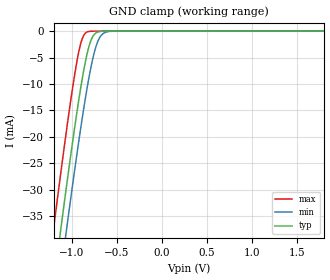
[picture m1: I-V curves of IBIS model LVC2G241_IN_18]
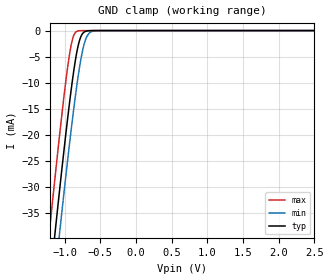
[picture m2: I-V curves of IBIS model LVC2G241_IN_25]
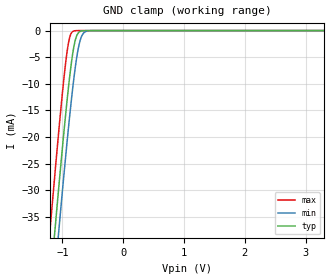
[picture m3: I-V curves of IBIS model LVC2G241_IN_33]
| TEXAS INSTRUMENTS INCORPORATED
| Standard Linear and Logic Group
| IBIS Model of SN74LVC2G241
| Dual Buffer/Driver with 3-State Outputs
| This file contains package information for the following:
|  TSSOP 8-pin (DCT) package as [Component] LVC2G241_DCT
|  VSSOP 8-pin (DCU) package as [Component] LVC2G241_DCU
|  NanoStar WCSP 8-pin (YEA) package as [Component] LVC2G241_YEA
|  NanoFree WCSP 8-pin (YZA) package as [Component] LVC2G241_YZA
|  NanoStar WCSP 8-pin (YEP) package as [Component] LVC2G241_YEP
|  NanoFree WCSP 8-pin (YZP) package as [Component] LVC2G241_YZP
| This device can be powered at the following Vccs:
| This device can be powered at the following Vccs:
|  1.8 volt Vcc
|  2.5 volt Vcc
|  3.3 volt Vcc
|  5 volt Vcc
| This file provides unique models under the [Model Selector] for each Vcc.
| For operation at a specific Vcc, select the appropriate model after each
| [Model Selector] keyword.
[IBIS Ver]   3.2
[Comment char]  |_char
[File Name]   sn74lvc2g241.ibs
[File Rev]   1.2 | d_die
[Date]   October 23, 2003
[Source]   Data created from TI-SPICE simulations at TI-SLL.
[Notes]   The following is an IBIS list for the LVC2G241.
   Please contact sllibis@ti.com with questions and
   comments concerning SLL IBIS models.
   -Power clamp data deleted as there is no power-clamp diode.
[Disclaimer] Property of Texas Instruments Incorporated.  Unauthorized
   reproduction and/or distribution is strictly prohibited.
   This product is protected under copyright law.
   Created  2002, (C) Copyright  2002, Texas Instruments
   Incorporated, All Rights Reserved
   UNLESS THERE IS A SIGNED, WRITTEN AGREEMENT TO THE
   CONTRARY, TEXAS INSTRUMENTS (TI) IS PROVIDING THE IBIS
   MODELS  AND WITHOUT ANY WARRANTY, EXPRESSED OR
   IMPLIED.  TI assumes no liability for:
   1) the accuracy of the IBIS models provided to your
   company;
   2) the proper functioning of these IBIS Models in your
   design or for any resulting applications; or
   3) infringement of patents, copyrights or intellectual
   property rights resulting from your use of these IBIS
   models.
   TI provides IBIS Models as a service to our customers.
   You and your company shall not distribute, sell or give
   these models to anyone else without prior written
   permission from TI.
   TI reserves the right to make changes to our products or
   to discontinue any semiconductor product or service
   without notice, and advises our customers to obtain the
   latest version of relevant information to verify, before
   placing orders, that the information being relied on is
   current.
   Please be aware that your receipt and use of the IBIS
   information provided shall serve as acceptance of these
   terms and conditions.  If you do not accept these terms,
   you should return or destroy the IBIS models and any
   other accompanying information immediately.
| Component LVC2G241_DCT 8-pin TSSOP
[Component]   LVC2G241_DCT
[Manufacturer]   Texas Instruments, Inc.
[Package]
|   typ   min   max
R_pkg   2.900e-02   2.800e-02   3.100e-02
L_pkg   1.796e-09   1.666e-09   1.924e-09
C_pkg   1.090e-13   8.300e-14   1.360e-13
[Pin]   signal_name   model_name   R_pin   L_pin   C_pin
1   1NOE   LVC2G241_IN   3.100e-02   1.894e-09   1.340e-13
2   1A   LVC2G241_IN   2.800e-02   1.697e-09   8.600e-14
3   2Y   LVC2G241_OUT   3.000e-02   1.722e-09   8.600e-14
4   GND   GND   3.000e-02   1.861e-09   1.300e-13
5   2A   LVC2G241_IN   2.800e-02   1.924e-09   1.360e-13
6   1Y   LVC2G241_OUT   2.900e-02   1.736e-09   8.600e-14
7   2OE   LVC2G241_IN   2.800e-02   1.666e-09   8.300e-14
8   VCC   POWER   3.000e-02   1.871e-09   1.320e-13
| Component LVC2G241_DCU 8-pin SOT
[Component]   LVC2G241_DCU
[Manufacturer]   Texas Instruments, Inc.
[Package]
|   typ   min   max
R_pkg   2.600e-02   2.300e-02   3.800e-02
L_pkg   1.394e-09   1.066e-09   2.046e-09
C_pkg   2.590e-13   2.150e-13   3.720e-13
[Pin]   signal_name   model_name   R_pin   L_pin   C_pin
1   1NOE   LVC2G241_IN   2.400e-02   1.520e-09   2.710e-13
2   1A   LVC2G241_IN   2.300e-02   1.112e-09   2.180e-13
3   2Y   LVC2G241_OUT   2.300e-02   1.070e-09   2.170e-13
4   GND   GND   2.700e-02   2.046e-09   3.720e-13
5   2A   LVC2G241_IN   2.700e-02   1.542e-09   2.730e-13
6   1Y   LVC2G241_IN   2.300e-02   1.100e-09   2.240e-13
7   2NOE   LVC2G241_OUT   2.300e-02   1.066e-09   2.150e-13
8   VCC   POWER   3.800e-02   1.696e-09   2.800e-13
| Component LVC2G241_YEA 8-pin NanoStar WCSP
[Component]   LVC2G241_YEA
[Manufacturer]   Texas Instruments, Inc.
[Package]
|   typ   min   max
R_pkg   0.001   0.001   0.001
L_pkg   0.021nH   0.021nH   0.021nH
C_pkg   0.043pF   0.042pF   0.044pF
[Pin]   signal_name   model_name   R_pin   L_pin   C_pin
1   1NOE   LVC2G241_IN   0.046   2.861nH   0.321pF
2   1A   LVC2G241_IN   0.037   2.437nH   0.286pF
3   2Y   LVC2G241_OUT   0.034   2.419nH   0.286pF
4   GND   GND   0.043   2.784nH   0.321pF
5   2A   LVC2G241_IN   0.043   2.784nH   0.321pF
6   1Y   LVC2G241_IN   0.035   2.420nH   0.286pF
7   2NOE   LVC2G241_OUT   0.037   2.437nH   0.286pF
8   VCC   POWER   0.046   2.860nH   0.321pF
| Component LVC2G241_YZA 8-pin NanoFree WCSP
[Component]   LVC2G241_YZA
[Manufacturer]   Texas Instruments, Inc.
[Package]
|   typ   min   max
R_pkg   0.001   0.001   0.001
L_pkg   0.021nH   0.021nH   0.021nH
C_pkg   0.043pF   0.042pF   0.044pF
[Pin]   signal_name   model_name   R_pin   L_pin   C_pin
1   1NOE   LVC2G241_IN   0.046   2.861nH   0.321pF
2   1A   LVC2G241_IN   0.037   2.437nH   0.286pF
3   2Y   LVC2G241_OUT   0.034   2.419nH   0.286pF
4   GND   GND   0.043   2.784nH   0.321pF
5   2A   LVC2G241_IN   0.043   2.784nH   0.321pF
6   1Y   LVC2G241_IN   0.035   2.420nH   0.286pF
7   2NOE   LVC2G241_OUT   0.037   2.437nH   0.286pF
8   VCC   POWER   0.046   2.860nH   0.321pF
| Component LVC2G241_YEP 8-pin NanoStar WCSP
[Component]   LVC2G241_YEP
[Manufacturer]   Texas Instruments, Inc.
[Package]
|   typ   min   max
R_pkg   0.001   0.001   0.001
L_pkg   0.021nH   0.021nH   0.021nH
C_pkg   0.043pF   0.042pF   0.044pF
[Pin]   signal_name   model_name   R_pin   L_pin   C_pin
1   1NOE   LVC2G241_IN   0.046   2.861nH   0.321pF
2   1A   LVC2G241_IN   0.037   2.437nH   0.286pF
3   2Y   LVC2G241_OUT   0.034   2.419nH   0.286pF
4   GND   GND   0.043   2.784nH   0.321pF
5   2A   LVC2G241_IN   0.043   2.784nH   0.321pF
6   1Y   LVC2G241_IN   0.035   2.420nH   0.286pF
7   2NOE   LVC2G241_OUT   0.037   2.437nH   0.286pF
8   VCC   POWER   0.046   2.860nH   0.321pF
| Component LVC2G241_YZP 8-pin NanoFree WCSP
[Component]   LVC2G241_YZP
[Manufacturer]   Texas Instruments, Inc.
[Package]
|   typ   min   max
R_pkg   0.001   0.001   0.001
L_pkg   0.021nH   0.021nH   0.021nH
C_pkg   0.043pF   0.042pF   0.044pF
[Pin]   signal_name   model_name   R_pin   L_pin   C_pin
1   1NOE   LVC2G241_IN   0.046   2.861nH   0.321pF
2   1A   LVC2G241_IN   0.037   2.437nH   0.286pF
3   2Y   LVC2G241_OUT   0.034   2.419nH   0.286pF
4   GND   GND   0.043   2.784nH   0.321pF
5   2A   LVC2G241_IN   0.043   2.784nH   0.321pF
6   1Y   LVC2G241_IN   0.035   2.420nH   0.286pF
7   2NOE   LVC2G241_OUT   0.037   2.437nH   0.286pF
8   VCC   POWER   0.046   2.860nH   0.321pF
| Model LVC2G241_IN
[Model Selector]   LVC2G241_IN
LVC2G241_IN_18   1.8 volt Vcc
LVC2G241_IN_25   2.5 volt Vcc
LVC2G241_IN_33   3.3 volt Vcc
LVC2G241_IN_50   5 volt Vcc
| Model LVC2G241_OUT
[Model Selector]   LVC2G241_OUT
LVC2G241_OUT_18   1.8 volt Vcc
LVC2G241_OUT_25   2.5 volt Vcc
LVC2G241_OUT_33   3.3 volt Vcc
LVC2G241_OUT_50   5 volt Vcc
| Models and submodels in the file (8): LVC2G241_IN_18 (Input), LVC2G241_IN_25 (Input), LVC2G241_IN_33 (Input), LVC2G241_IN_50 (Input), LVC2G241_OUT_18 (3-state), LVC2G241_OUT_25 (3-state), LVC2G241_OUT_33 (3-state), LVC2G241_OUT_50 (3-state)
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[Model]   LVC2G241_IN_18
Model_type  Input
Vinl=0.5775
Vinh=1.2675
| variable   typ   min   max
C_comp   3.50pF   2.99pF   4.32pF
[Temperature Range]   40   100   -40
| Ambient temperature   25   85   -40
[Voltage range]   1.8   1.65   1.95
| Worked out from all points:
|   GND clamp passes 1 mA (typ) near -0.77 V on its own axis
[GND Clamp]
| LVC2G241D_IN_18
|   Voltage   I(typ)   I(min)   I(max)
-1.8V     -129.8mA   -137.8mA   -119.7mA
-1.205V   -48.27mA   -56.56mA   -37.63mA
-1.125V   -37.77mA   -46.06mA   -27.13mA
-1.06V    -29.44mA   -37.69mA   -18.89mA
-980mV    -19.61mA   -27.69mA   -9.485mA
-925mV    -13.29mA   -21.11mA   -4.122mA
-880mV    -8.606mA   -15.99mA   -1.263mA
-835mV    -4.656mA   -11.25mA   -214.1uA
-780mV    -1.472mA   -6.227mA   -17.15uA
-725mV    -285.9uA   -2.596mA   -1.294uA
-615mV    -6.479uA   -167.8uA   -7.305nA
1.8V      3.326pA    6.142pA    3.026pA
[Model]   LVC2G241_IN_25
Model_type  Input
Vinl=0.7
Vinh=1.7
| variable   typ   min   max
C_comp   3.42pF   2.80pF   4.39pF
[Temperature Range]   40   100   -40
| Ambient temperature   25   85   -40
[Voltage range]   2.5   2.3   2.7
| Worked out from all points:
|   GND clamp passes 1 mA (typ) near -0.77 V on its own axis
[GND Clamp]
| LVC2G241D_IN_25
|   Voltage   I(typ)   I(min)   I(max)
-2.5V     -228.1mA   -235.8mA   -218.5mA
-1.23V    -51.59mA   -59.87mA   -40.97mA
-1.2V     -47.61mA   -55.9mA    -36.97mA
-1.13V    -38.42mA   -46.71mA   -27.77mA
-1.07V    -30.71mA   -38.96mA   -20.13mA
-925mV    -13.29mA   -21.11mA   -4.122mA
-880mV    -8.606mA   -15.99mA   -1.263mA
-830mV    -4.281mA   -10.75mA   -171.6uA
-780mV    -1.472mA   -6.227mA   -17.15uA
-720mV    -242.5uA   -2.354mA   -1.023uA
-600mV    -3.832uA   -109.2uA   -3.608nA
2.5V      4.713pA    7.577pA    4.389pA
[Model]   LVC2G241_IN_33
Model_type  Input
Vinl=0.8
Vinh=2.0
| variable   typ   min   max
C_comp   3.34pF   2.68pF   4.36pF
[Temperature Range]   40   100   -40
| Ambient temperature   25   85   -40
[Voltage range]   3.3   3   3.6
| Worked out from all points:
|   GND clamp passes 1 mA (typ) near -0.77 V on its own axis
[GND Clamp]
| LVC2G241D_IN_33
|   Voltage   I(typ)   I(min)   I(max)
-3.3V     -341.5mA   -348.9mA   -332.3mA
-1.215V   -49.6mA    -57.88mA   -38.96mA
-1.185V   -45.62mA   -53.91mA   -34.98mA
-1.125V   -37.77mA   -46.06mA   -27.13mA
-1.065V   -30.08mA   -38.33mA   -19.51mA
-920mV    -12.75mA   -20.53mA   -3.718mA
-875mV    -8.124mA   -15.45mA   -1.065mA
-825mV    -3.922mA   -10.26mA   -137.1uA
-775mV    -1.291mA   -5.83mA    -13.57uA
-715mV    -205.4uA   -2.128mA   -808.5nA
-585mV    -2.266uA   -70.82uA   -1.783nA
3.3V      6.304pA    9.258pA    5.93pA
